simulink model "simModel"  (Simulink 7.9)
settings: Solver=ode15s  StartTime=0.0  StopTime=stopTime  MaxStep=0.1  RelTol=1e-3
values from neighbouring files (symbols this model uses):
  dTime = 20    [mainStepResponsePlotPo.m]
  ysTime = 1    [mainStepResponsePlotPo.m]
libraries: cstblocks x2

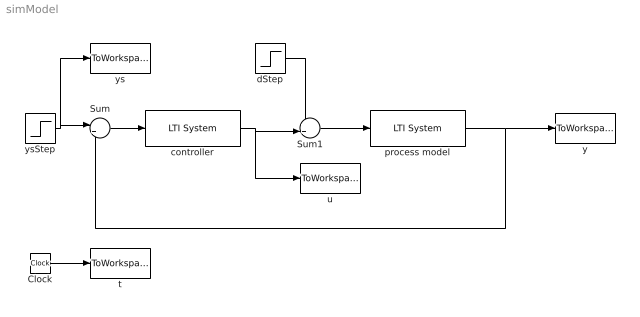
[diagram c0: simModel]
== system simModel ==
  Clock : Clock
  Sum : Sum  Inputs=|+-
  Sum1 : Sum  Inputs=++|
  controller : cstblocks/LTI System  sys=gc  IC=[]
  dStep : Step  Time=dTime  SampleTime=0
  process model : cstblocks/LTI System  sys=gp  IC=[]
  t : ToWorkspace  VariableName=t  SampleTime=-1
  u : ToWorkspace  VariableName=u  SampleTime=-1
  y : ToWorkspace  VariableName=y  SampleTime=-1
  ys : ToWorkspace  VariableName=ys  SampleTime=-1
  ysStep : Step  Time=ysTime  SampleTime=0
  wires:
  ysStep/1 -> Sum/1, ys/1
  Sum/1 -> controller/1
  controller/1 -> Sum1/2, u/1
  Sum1/1 -> process model/1
  dStep/1 -> Sum1/1
  process model/1 -> Sum/2, y/1
  Clock/1 -> t/1
